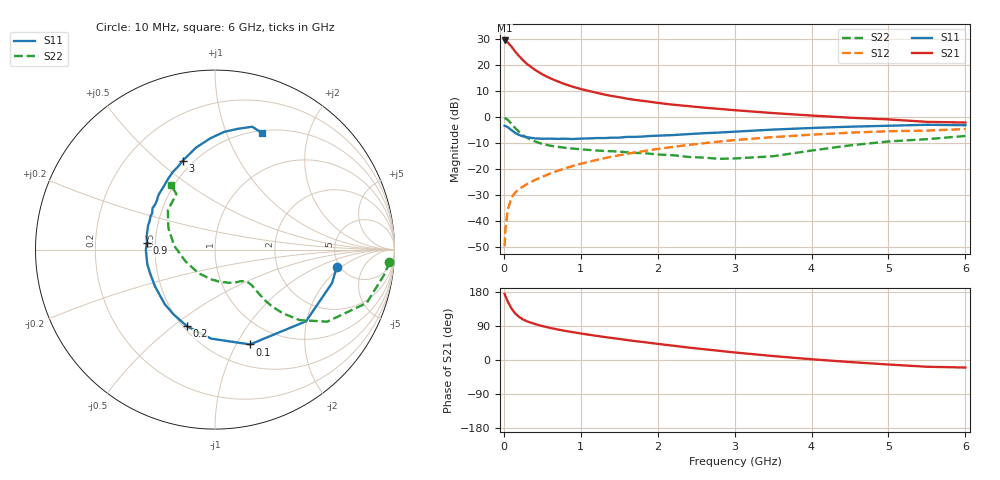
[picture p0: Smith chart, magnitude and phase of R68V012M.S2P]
! SIEMENS Small Signal Semiconductors
! BFR193
! Si NPN RF Bipolar Junction Transistor in SOT23
! VCE = 8 V  IC = 12 mA
! Common Emitter S-Parameters:  May  1996
# GHz  S  MA  R  50
!  f  S11  S21  S12  S22
! GHz  MAG  ANG  MAG  ANG  MAG  ANG  MAG  ANG
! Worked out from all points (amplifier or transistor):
!   36 points, 10 MHz to 6 GHz, reference 50 ohm
!   highest |S21| = 29.5 dB at 10 MHz (marker M1)
!   |S21| within 3 dB of that: start of sweep to 115.2 MHz
!   unconditionally stable (mu >= 1): 730.6 MHz to 2.03 GHz
!   at 250 MHz: K = 0.68, MSG = 24.3 dB, |S12| = -26.7 dB
!   at 1.4 GHz: K = 1.03, MAG = 10.6 dB, |S12| = -15.2 dB
!   at 6 GHz: K = 0.94, MSG = 1.3 dB, |S12| = -4.6 dB
!   S11 on the Smith chart (normalised r, x): 10 MHz: 4.71, -1.72; 100 MHz: 0.74, -1.14; 200 MHz: 0.52, -0.56; 900 MHz: 0.45, +0.04; 3 GHz: 0.44, +0.60; 6 GHz: 0.53, +1.35
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0.01  0.6855 -8.1  30 174.4  0.0033 86.4  0.9742 -4.1
0.02  0.6784 -15.9  29.3 169.1  0.0069 82.7  0.9547 -8.2
0.05  0.6455 -38.2  27.6 154.6  0.0164 73.6  0.8958 -19.4
0.1  0.5633 -69.7  22.77 135.6  0.0285 63.6  0.7431 -32.7
0.15  0.4966 -92.4  18.11 122.3  0.0359 58.8  0.6135 -39.8
0.2  0.4545 -110.2  14.91 113.5  0.0415 57.9  0.5179 -43.2
0.25  0.4281 -123.0  12.45 106.9  0.0464 57.5  0.448 -44.9
0.3  0.4127 -132.9  10.64 102.3  0.0514 58.5  0.4031 -45.4
0.4  0.3921 -148.4  8.258 95.3  0.0616 60.1  0.3442 -45.1
0.5  0.3852 -159.0  6.69 89.5  0.0712 62.0  0.3054 -44.5
0.6  0.3861 -167.3  5.646 84.8  0.0823 63.1  0.2838 -44.2
0.7  0.3837 -174.8  4.887 80.5  0.093 63.9  0.2695 -44.4
0.9  0.3804 174.3  3.848 73.3  0.1157 64.1  0.2487 -45.4
1.1  0.3904 164.9  3.212 66.9  0.1383 63.9  0.2351 -48.5
1.3  0.3967 156.8  2.747 60.9  0.1617 62.7  0.2244 -51.9
1.6  0.4179 146.4  2.277 52.7  0.1968 60.3  0.2116 -59.4
2.2  0.453 129.2  1.742 37.8  0.2686 54.1  0.1858 -79.5
3  0.5268 110.0  1.366 19.9  0.3629 43.5  0.1608 -124.2
3.5  0.5782 100.5  1.201 10.4  0.4139 36.0  0.1774 -158.7
4.5  0.6574 85.7  0.979 -5.4  0.5043 21.5  0.2871 154.9
5.5  0.7151 73.2  0.814 -17.8  0.5531 6.6  0.3779 124.7
6  0.7011 67.9  0.79 -19.9  0.591 2.2  0.4353 124.4
